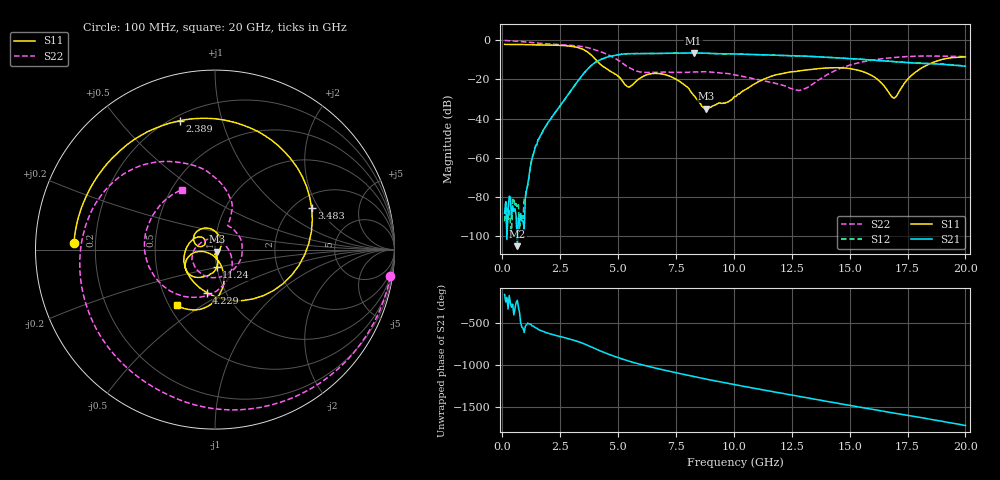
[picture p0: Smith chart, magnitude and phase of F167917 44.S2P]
!  2-Port S-parameters saved by WinCal
! VAR MeasName=S-Parameters (CALIBRATED_DATA) read from VNA (N5242A)
! VAR MeasDate=2016-11-22 9:01:57
! VAR NAME=F167917 44
! VAR FILENAME=F167917 44.S2P
! VAR DATE=2016-11-22 9:01:57
! VAR PHYS_PORTS=1,2
# Hz S DB R 50
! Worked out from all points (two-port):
!   401 points, 100 MHz to 20 GHz, reference 50 ohm
!   highest |S21| = -6.45 dB at 8.259 GHz (marker M1); lowest = -105.2 dB at 647.2 MHz (marker M2)
!   |S21| within 3 dB of the highest: 4.342 GHz to 15.12 GHz (10.78 GHz wide, 111 % of centre)
!   lowest |S11| = -35.0 dB at 8.806 GHz (marker M3), VSWR 1.04, Z = 51.3 - j1.24 ohm
!   |S11| at or under -10 dB: 4.043 GHz to 18.93 GHz (14.89 GHz wide, 130 % of centre)
!   |S22| runs from -25.6 to -0.1 dB; largest |S21 - S12| = 0.0063
!   S11 on the Smith chart (normalised r, x): 100 MHz: 0.12, +0.02; 2.389 GHz: 0.23, +0.74; 3.483 GHz: 2.47, +1.73; 4.229 GHz: 0.82, -0.42; 11.24 GHz: 1.00, -0.20; 20 GHz: 0.55, -0.40
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1e8  -2.09 177.3  -88.41 -153.6  -92.53 81.5  -0.10 -8.7
6.4725e8  -2.16 162.8  -105.16 136.3  -85.38 -155.4  -0.49 -52.2
9.955e8  -2.22 153.3  -80.68 -174.3  -79.47 -147.8  -0.83 -77.4
1.493e9  -2.31 138.7  -53.30 161.4  -53.37 162.2  -1.43 -109.2
2.3885e9  -2.56 105.1  -35.23 68.3  -35.21 68.1  -2.14 -156.5
3.43325e9  -4.39 28.9  -18.19 -15.3  -18.20 -15.3  -3.18 151.0
3.483e9  -4.65 23.1  -17.46 -20.6  -17.46 -20.5  -3.27 148.3
3.881e9  -8.01 -35.0  -12.51 -67.9  -12.47 -67.8  -4.40 127.0
4.22925e9  -12.25 -101.0  -9.99 -110.9  -9.95 -110.9  -5.79 110.0
5.12475e9  -19.74 137.4  -7.19 157.0  -7.20 156.9  -11.04 70.6
5.871e9  -19.98 168.0  -6.81 93.8  -6.80 93.7  -15.95 63.0
6.7665e9  -17.02 128.9  -6.71 32.4  -6.72 32.1  -16.34 38.8
8.259e9  -28.03 31.5  -6.45 -58.9  -6.48 -58.7  -16.17 -70.6
8.80625e9  -35.00 -42.6  -6.66 -90.6  -6.66 -90.7  -16.06 -108.0
1.005e10  -28.72 -79.6  -7.02 -157.5  -7.03 -157.4  -17.74 -166.4
1.1244e10  -20.12 -84.5  -7.42 140.9  -7.40 141.2  -20.60 161.1
1.338325e10  -14.85 -121.2  -8.28 33.6  -8.23 33.6  -22.56 1.1
1.55225e10  -15.83 -162.4  -9.75 -71.3  -9.76 -71.7  -11.13 -107.5
1.67165e10  -27.19 -156.6  -10.69 -129.0  -10.76 -128.7  -9.02 -146.1
1.696525e10  -29.19 -109.1  -11.00 -141.0  -10.93 -140.4  -8.74 -153.6
1.835825e10  -12.56 -81.8  -11.91 153.6  -11.77 153.9  -8.01 165.7
2e10  -8.49 -124.4  -13.21 72.5  -13.07 72.1  -8.40 118.8
